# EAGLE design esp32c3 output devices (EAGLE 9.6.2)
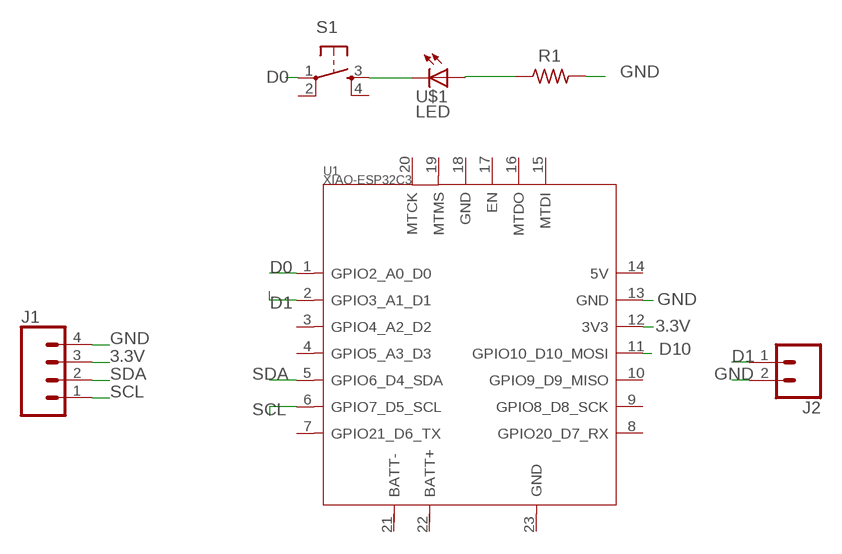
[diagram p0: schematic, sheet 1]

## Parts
J1  CONN_04PAD  [1X04_SOLDER_PADS]
J2  CONN_02PAD  [1X02_SOLDER_PADS]
R1  RES-US1206  [R1206]
S1  6MM_SWITCH6MM_SWITCH  [6MM_SWITCH]
U1  XIAO-ESP32C3  [XIAO-ESP32C3-MODULE14P-2.54-21X17.8MM]
U$1  LED  [LED1206]

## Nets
3.3V: J1.3 U1.12(3V3)
D0: S1.1(P) U1.1(GPIO2_A0_D0)
D1: J2.1 U1.2(GPIO3_A1_D1)
D10: U1.11(GPIO10_D10_MOSI)
GND: J1.4 J2.2 R1.2 U1.13(GND)
LED: S1.3(S) U$1.2(C)
N$6: R1.1 U$1.1(A)
SCL: J1.1 U1.6(GPIO7_D5_SCL)
SDA: J1.2 U1.5(GPIO6_D4_SDA)
Unconnected: S1.2(P1) S1.4(S1) U1.3(GPIO4_A2_D2) U1.4(GPIO5_A3_D3) U1.7(GPIO21_D6_TX) U1.8(GPIO20_D7_RX) U1.9(GPIO8_D8_SCK) U1.10(GPIO9_D9_MISO) U1.14(5V) U1.15(MTDI) U1.16(MTDO) U1.17(EN) U1.18(GND) U1.19(MTMS) U1.20(MTCK) U1.21(BATT-) U1.22(BATT+) U1.23(GND)

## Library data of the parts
J1 = 4 pin C:CONN_04: Multi connection point. Often used as Generic Header-pin footprint for 0.1 inch spaced/style header connections On any of the 0.1 inch spaced packages, you can populate with these: Break Away Headers - Straight (PRT-00116) Break Away Male Headers - Right Angle (PRT-00553) Female Headers (PRT-00115)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
J2 = 2 pin C:CONN_02: Multi connection point. Often used as Generic Header-pin footprint for 0.1 inch spaced/style header connections
R1 = fab:RES-US: Resistor (US Symbol)
S1 = fab:6MM_SWITCH: OMRON SWITCH
U1 = Seeed Studio XIAO Series ESP32 C3:XIAO-ESP32C3: Seeed Studio XIAO ESP32C3 - Espressif ESP32-C3 WiFi BLE Microcontroller - 32-bit 160MHz RISC-V processor Seeed SKU: 113991054 Seeed Studio XIAO ESP32C3 featuring ESP32C3 carries a complete Wi-Fi system along with Bluetooth Low Energy function. With its exquisite design, WiFi+BT ability, it's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
U$1 = fab:LED: LED

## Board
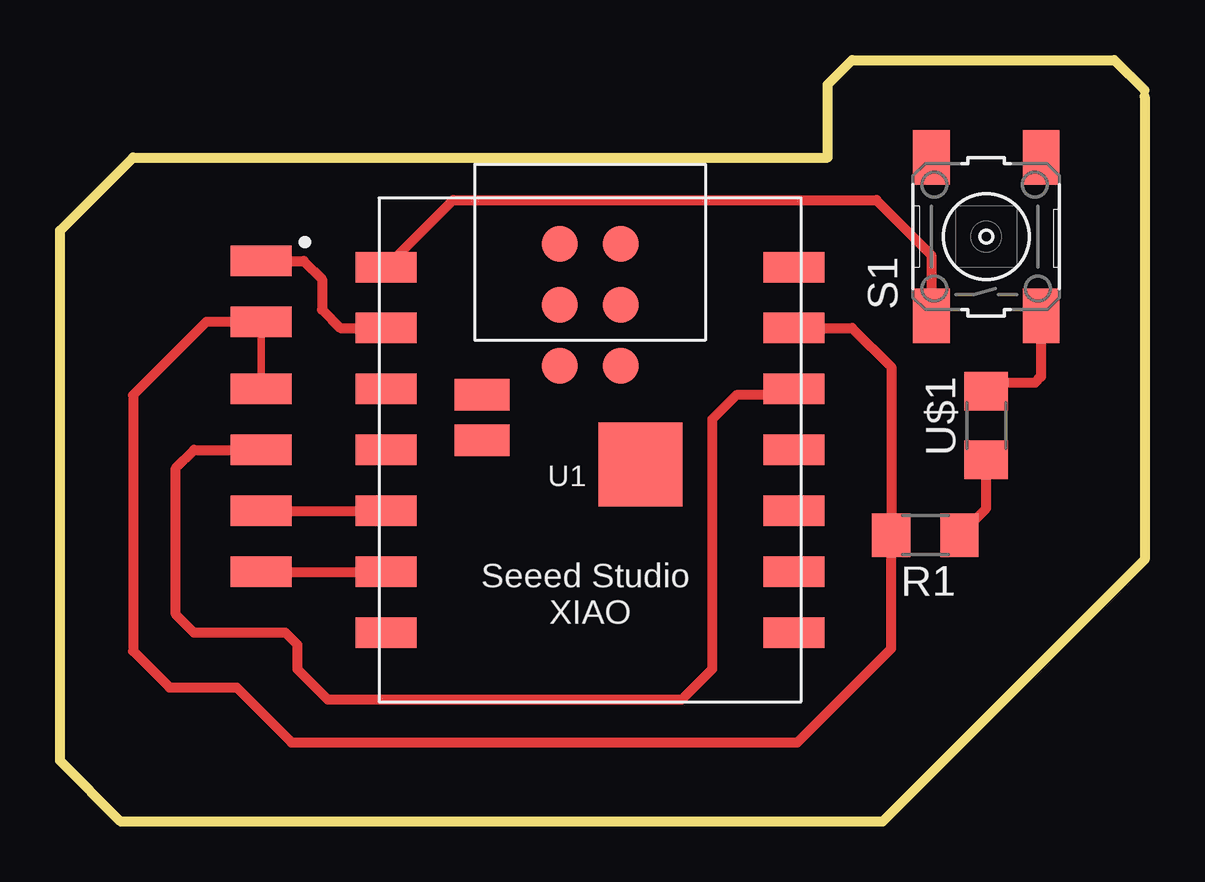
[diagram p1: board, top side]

Size 45.21 x 31.75 mm. Coordinates in mm from the lower left corner, seen from the top.
Outline: 45.21,30.48 43.94,31.75 33.02,31.75 32,30.73 32,27.69 3.05,27.69 0,24.64 0,2.54 2.54,0 34.29,0 45.21,10.92 45.21,30.23
Copper layers (1*16): Top 0.035mm / dielectric 0.15mm / Bottom 0.035mm
Design rules "default": minimum track width 6mil, minimum drill 0.35mm, track to track 6mil, track to pad 6mil, pad to pad 6mil, via to via 6mil, smd to smd 6mil, copper to edge 40mil, drill to drill 6mil, minimum pad ring 10mil, minimum via ring 8mil, stop-mask expansion 4mil, vias tented up to drill 0mil, thermal gap 10mil

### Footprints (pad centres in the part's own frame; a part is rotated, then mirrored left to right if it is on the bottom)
1X04_SOLDER_PADS = smd 2.54 x 1.27: 1 0,2.54; 2 0,5.08; 3 0,7.62; 4 0,10.16
1X02_SOLDER_PADS = smd 2.54 x 1.27: 1 0,2.54; 2 0,0
R1206 = smd 1.6 x 1.803: 1 -1.422,0; 2 1.422,0
6MM_SWITCH = smd 2.286 x 1.524: 1 -3.302,2.286; 2 3.302,2.286; 3 -3.302,-2.286; 4 3.302,-2.286
XIAO-ESP32C3-MODULE14P-2.54-21X17.8MM = smd 2.54 x 1.27: 1 -8.5,7.62; 2 -8.5,5.08; 3 -8.5,2.54; 4 -8.5,0; 5 -8.5,-2.54; 6 -8.5,-5.08; 7 -8.5,-7.62; 8 8.5,-7.62; 9 8.5,-5.08; 10 8.5,-2.54; 11 8.5,0; 12 8.5,2.54; 13 8.5,5.08; 14 8.5,7.62 | smd 1.5 x 1.5: 15 -1.27,8.58; 16 1.27,8.58; 17 -1.27,6.04; 18 1.27,6.04; 19 -1.27,3.5; 20 1.27,3.5 | smd 2.3 x 1.3: 21 -4.5,2.3; 22 -4.5,0.4 | smd 3.5 x 3.5: 23 2.1,-0.6
LED1206 = smd 1.6 x 1.803: 1 -1.422,0; 2 1.422,0

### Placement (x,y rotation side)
J1  8.38,7.87 0 top
J2  8.38,20.83 0 top
R1  36.07,11.94 180 top
S1  38.61,24.38 90 top
U1  22.1,15.49 0 top
U$1  38.61,16.51 90 top

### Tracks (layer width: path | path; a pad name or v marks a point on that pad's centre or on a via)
3.3V
  Top 0.406: 29.72,18.03 U1.12 30.34,17.78 28.19,17.78 27.18,16.76 27.18,6.35 25.91,5.08 11.18,5.08 9.91,6.35 9.91,7.37 9.4,7.87 5.59,7.87 4.83,8.64 4.83,14.73 5.59,15.49 J1.3
D0
  Top 0.305: 36.32,21.59 36.32,21.34 S1.1
  Top 0.406: U1.1 16.39,25.91 34.04,25.91 36.32,23.62 36.32,21.34
D1
  Top 0.406: J2.1 10.16,23.37 10.92,22.61 10.92,21.34 11.68,20.57 U1.2
GND
  Top 0.305: J1.4 8.13,18.03 8.38,18.29 J2.2
  Top 0.406: J2.2 6.1,20.83 3.05,17.78 3.05,7.11 4.57,5.59 7.37,5.59 9.65,3.3 30.73,3.3 34.65,7.21 R1.2 34.65,18.95 33.02,20.57 U1.13
LED
  Top 0.305: 40.89,20.22 S1.3
  Top 0.406: 39.27,17.93 U$1.2 38.61,18.54 38.86,18.29 40.64,18.29 40.89,18.54 S1.3
N$6
  Top 0.406: R1.1 38.61,13.06 U$1.1
SCL
  Top 0.406: J1.1 U1.6
SDA
  Top 0.406: J1.2 U1.5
